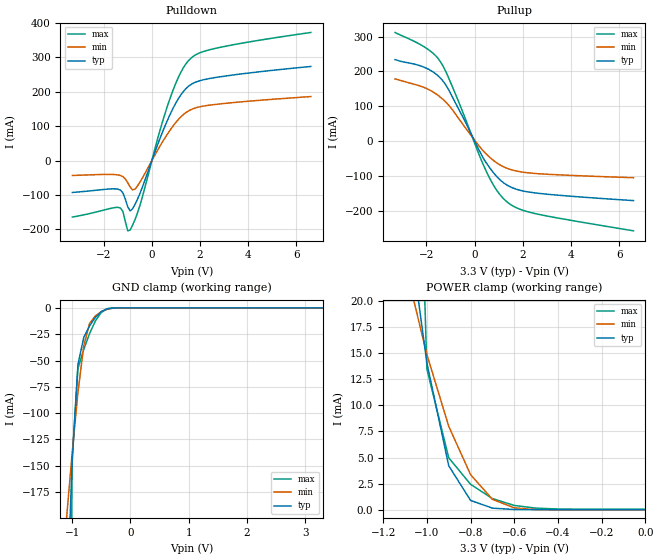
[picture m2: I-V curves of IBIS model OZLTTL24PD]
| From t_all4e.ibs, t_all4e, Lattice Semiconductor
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|   OZLTTL24PD
[Model]   OZLTTL24PD
Model_type   3-state
Polarity   Non-Inverting
Enable   Active-Low
C_comp   2pF   2pF   2pF
[Temperature Range]   25.0000   125.0000   -40.0000
[Voltage Range]   3.3000V   3.0000V   3.6000V
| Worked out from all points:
|   slope of the pulldown table from 0 to 0.495 V, typ, clamps not added: 5.38 ohm
|   slope of the pullup table from 0 to 0.495 V, typ, clamps not added: 7.79 ohm
|   GND clamp passes 1 mA (typ) near -0.40 V on its own axis
|   POWER clamp passes 1 mA (typ) near -0.80 V on its own axis
[Pulldown]
|voltage   I(typ)   I(min)   I(max)
-3.3V     -92.63mA   -43.21mA   -164.1mA
-1.4V     -83.18mA   -41.77mA   -135.9mA
-1.2V     -93.88mA   -46.78mA   -148.2mA
-1V       -134.4mA   -64.53mA   -204.3mA
-900mV    -146.4mA   -77mA      -201.8mA
-600mV    -112.8mA   -74.16mA   -152.9mA
300mV     57.56mA    37.7mA     78.81mA
800mV     140.6mA    92.96mA    189.8mA
1.3V      200.3mA    133.5mA    269.1mA
1.7V      224.5mA    150.6mA    302.3mA
2.9V      244.5mA    165.5mA    330.5mA
6.6V      273.9mA    186.3mA    372.7mA
[Pullup]
|voltage   I(typ)   I(min)   I(max)
-3.3V     234.1mA    178.5mA    312mA
-2V       209.4mA    151.3mA    266.7mA
-1.6V     192.5mA    135.6mA    244.2mA
-1.4V     179.8mA    125.1mA    226.2mA
-1.1V     150.4mA    105.2mA    185.4mA
-800mV    110.5mA    78.55mA    136.3mA
500mV     -64.13mA   -38.05mA   -88.87mA
900mV     -100.3mA   -61.56mA   -139.3mA
1.3V      -124.3mA   -76.81mA   -171.9mA
1.7V      -137.5mA   -85.45mA   -190.3mA
2.4V      -147.8mA   -92.32mA   -206.4mA
6.6V      -171mA     -105.2mA   -257.9mA
[GND_clamp]
|voltage   I(typ)   I(min)   I(max)
-3.3V     -4.405A    -1.803A    -40.47A
-1.1V     -296.4mA   -202.8mA   -979.3mA
-1V       -147.6mA   -138.6mA   -143.7mA
-900mV    -53.79mA   -80.42mA   -57.6mA
-800mV    -28.05mA   -35.98mA   -39.41mA
-700mV    -17.1mA    -14.8mA    -24.33mA
-600mV    -8.999mA   -7.523mA   -12.36mA
-500mV    -3.595mA   -3.617mA   -4.359mA
-400mV    -879.9uA   -1.324mA   -818.8uA
-300mV    -134.5uA   -303.4uA   -113.2uA
3.3V      27.16uA    10.44uA    65.22uA
[POWER_clamp]
|voltage   I(typ)   I(min)   I(max)
-3.3V     682mA      379.6mA    3.878A
-1.1V     29.47mA    23.43mA    82.94mA
-1V       14.05mA    14.85mA    13.46mA
-900mV    4.218mA    7.985mA    4.978mA
-800mV    910uA      3.369mA    2.448mA
-700mV    172.8uA    1.011mA    1.084mA
-600mV    39.84uA    197.6uA    429.9uA
-500mV    27.92uA    30.49uA    170.3uA
-400mV    27.27uA    11.82uA    89.74uA
0V        27.16uA    10.3uA     65.38uA
[Ramp]
| variable   typ   min   max
dV/dt_r   1.7021/0.3465ns   1.3998/1.0389ns   1.9655/0.1535ns
dV/dt_f   1.7950/0.5692ns   1.5442/1.2795ns   2.0177/0.2629ns
